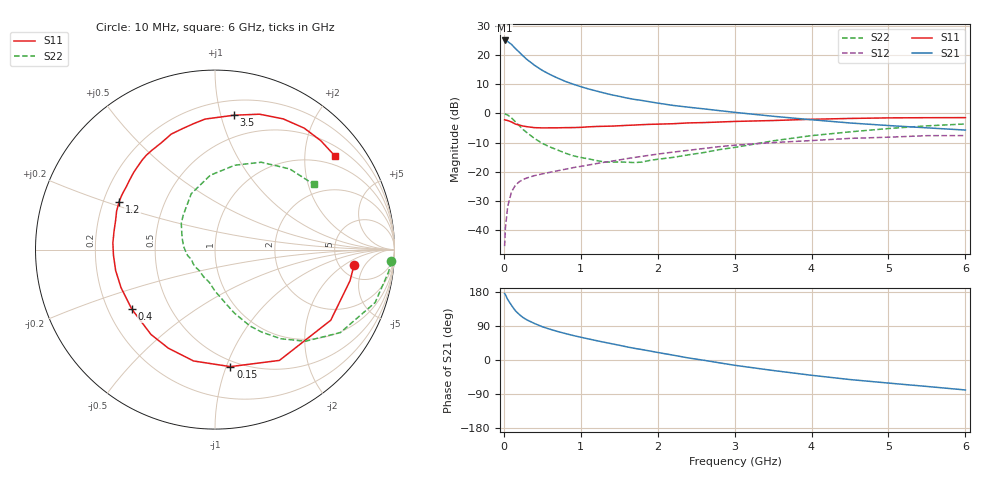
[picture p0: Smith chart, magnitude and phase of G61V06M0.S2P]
! SIEMENS Small Signal Semiconductors
! BFG193
! Si NPN RF Bipolar Junction Transistor in SOT223
! VCE = 1 V  IC = 6 mA
! Common Emitter S-Parameters:  August  1996
# GHz  S  MA  R  50
!  f  S11  S21  S12  S22
! GHz  MAG  ANG  MAG  ANG  MAG  ANG  MAG  ANG
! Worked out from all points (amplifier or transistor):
!   36 points, 10 MHz to 6 GHz, reference 50 ohm
!   highest |S21| = 25.1 dB at 10 MHz (marker M1)
!   |S21| within 3 dB of that: start of sweep to 158.5 MHz
!   unconditionally stable (mu >= 1): 984.9 MHz to 2.985 GHz
!   at 250 MHz: K = 0.39, MSG = 21.3 dB, |S12| = -22.7 dB
!   at 1.4 GHz: K = 1.10, MAG = 9.5 dB, |S12| = -16.4 dB
!   at 6 GHz: K = 0.97, MSG = 0.9 dB, |S12| = -7.6 dB
!   S11 on the Smith chart (normalised r, x): 10 MHz: 6.72, -2.98; 150 MHz: 0.45, -1.03; 400 MHz: 0.30, -0.29; 1.2 GHz: 0.27, +0.22; 3.5 GHz: 0.31, +1.10; 6 GHz: 0.74, +2.74
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0.01  0.7794 -6.4  18.07 175.7  0.0052 87.7  0.9846 -3.8
0.02  0.772 -13.0  17.94 172.5  0.0105 85.8  0.9747 -7.4
0.05  0.7555 -31.4  17.3 159.7  0.0251 74.2  0.9396 -18.3
0.1  0.7142 -59.8  15.45 144.1  0.045 62.5  0.8377 -33.5
0.15  0.6577 -82.5  13.1 129.9  0.058 52.4  0.7171 -45.4
0.2  0.6319 -100.9  11.36 120.3  0.0668 47.7  0.6181 -53.5
0.25  0.6077 -115.3  9.776 112.0  0.0732 43.0  0.5293 -60.4
0.3  0.5924 -127.0  8.515 105.8  0.0777 40.2  0.4681 -65.4
0.4  0.57 -144.5  6.743 96.2  0.0853 37.3  0.3702 -73.0
0.5  0.5649 -157.9  5.518 87.8  0.0912 36.1  0.3062 -78.7
0.6  0.5657 -168.1  4.688 81.2  0.0972 35.9  0.2649 -83.9
0.7  0.5665 -176.7  4.062 75.2  0.1034 35.9  0.2345 -89.3
0.9  0.5718 169.6  3.197 64.7  0.1169 35.8  0.1872 -99.2
1.1  0.5887 158.6  2.645 55.6  0.1295 35.6  0.1654 -111.9
1.2  0.5974 153.5  2.442 51.3  0.137 35.5  0.1555 -118.5
1.6  0.6243 136.6  1.843 34.6  0.1671 32.0  0.1451 -146.4
2.2  0.6663 116.6  1.377 12.8  0.2163 23.7  0.1755 174.2
2.8  0.7128 99.3  1.12 -7.4  0.2685 12.9  0.2385 142.0
3.5  0.7563 81.9  0.896 -27.7  0.3157 -2.9  0.3384 113.0
4.5  0.8214 62.5  0.686 -51.6  0.3727 -22.1  0.4828 76.8
5.5  0.846 45.8  0.566 -69.8  0.415 -45.3  0.6126 47.2
6  0.8478 37.9  0.518 -79.1  0.4165 -58.6  0.6598 33.4
